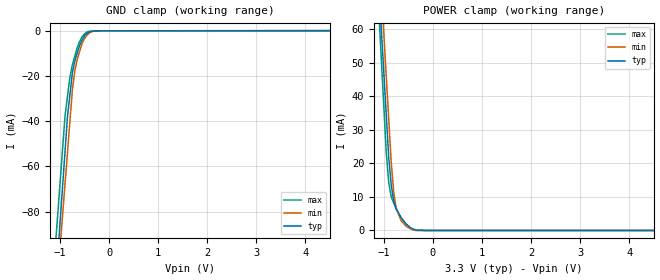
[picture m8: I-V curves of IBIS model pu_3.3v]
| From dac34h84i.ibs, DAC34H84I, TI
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[Model] pu_3.3v
Model_type Input
Vinl = 990.000mV
Vinh = 2.31000V
C_comp 609.000fF 588.000fF 630.000fF
| variable typ   min   max
[Voltage Range] 3.30000V 3.00000V 3.60000V
[POWER Clamp Reference] 3.30000V 3.00000V 3.60000V
[GND Clamp Reference] 0.00000V 0.00000V 0.00000V
[Temperature Range] 25   125   -40
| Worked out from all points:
|   GND clamp passes 1 mA (typ) near -0.44 V on its own axis
|   POWER clamp passes 1 mA (typ) near -0.47 V on its own axis
[GND Clamp]
-3.3V     -798.7mA   -735.1mA   -740.2mA
-900mV    -53.61mA   -67.96mA   -37.82mA
-850mV    -38.09mA   -54.06mA   -29.18mA
-800mV    -28.39mA   -40.16mA   -20.55mA
-750mV    -18.7mA    -26.27mA   -15.03mA
-700mV    -13.36mA   -17.74mA   -11.24mA
-650mV    -9.904mA   -12.53mA   -7.454mA
-550mV    -3.991mA   -5.523mA   -2.621mA
-450mV    -1.131mA   -1.891mA   -566.3uA
-350mV    -182.4uA   -406uA     -164.4uA
-150mV    -26.84uA   -24.75uA   -32.78uA
6.6V      49.82uA    64.96uA    34.03uA
[POWER Clamp]
-3.3V     629.5mA    645mA      672.2mA
-1.15V    84.93mA    96.82mA    78.27mA
-1.05V    59.6mA     71.32mA    50.65mA
-950mV    34.27mA    45.83mA    23.02mA
-900mV    21.61mA    33.08mA    14.24mA
-850mV    13.64mA    20.33mA    10.08mA
-800mV    8.872mA    11.61mA    8.258mA
-750mV    6.517mA    6.669mA    6.432mA
-650mV    3.865mA    2.963mA    3.805mA
-550mV    2.006mA    1.352mA    1.905mA
-400mV    456uA      132.3uA    239.3uA
6.6V      0A         0A         0A
